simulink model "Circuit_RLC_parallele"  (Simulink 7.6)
settings: Solver=ode23t  StartTime=0.0  StopTime=0.05  RelTol=1e-3
InitFcn:
  | clc
  | clear all
  | delete *.mat
StopFcn:
  | close all
  | load circuit_RLC_parallele.mat
  | plot(x(1,:),x(2,:),x(1,:),x(3,:))
  | grid
  | title('Courant, tension - Circuit RLC parallèle')
  | xlabel('temps')
  | axis([0 0.05 -1 2])
libraries: powerlib x10

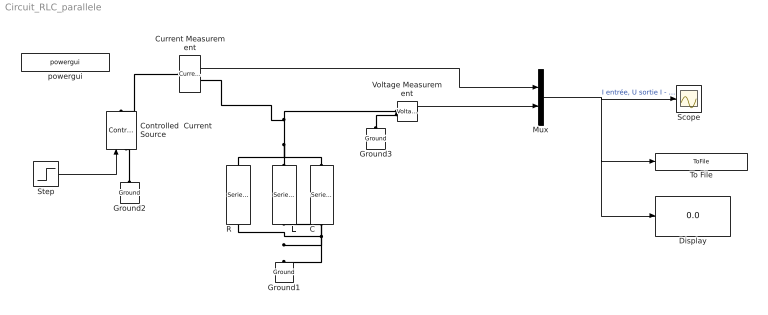
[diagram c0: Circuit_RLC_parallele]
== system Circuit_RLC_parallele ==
  C : powerlib/Elements/Series RLC Branch  DialogController=POWERSYS.PowerSysDialog  PhysicalDomain=powersysdomain  SubClassName=unknown  LeftPortType=p1  RightPortType=p1  LConnTagsString=__new0  RConnTagsString=__new0  BranchType=C  Resistance=1  Inductance=1e-3  SetiL0=off  InitialCurrent=0  Capacitance=0.001  Setx0=off  InitialVoltage=0  Measurements=None
  Controlled  Current Source : powerlib/Electrical Sources/Controlled Current Source  DialogController=POWERSYS.PowerSysDialog  SystemSampleTime=-1  Initialize=on  Source_Type=AC  Amplitude=0  Phase=0  Frequency=0  Measurements=None
  Current Measurement : powerlib/Measurements/Current Measurement  DialogController=POWERSYS.PowerSysDialog  SystemSampleTime=-1  PhasorSimulation=off  OutputType=Complex  PSBequivalent=0
  Display : Display
  Ground1 : powerlib/Elements/Ground  DialogController=POWERSYS.PowerSysDialog  PhysicalDomain=powersysdomain  SubClassName=unknown  LeftPortType=p1  RightPortType=p1  LConnTagsString=a
  Ground2 : powerlib/Elements/Ground  DialogController=POWERSYS.PowerSysDialog  PhysicalDomain=powersysdomain  SubClassName=unknown  LeftPortType=p1  RightPortType=p1  LConnTagsString=a
  Ground3 : powerlib/Elements/Ground  DialogController=POWERSYS.PowerSysDialog  PhysicalDomain=powersysdomain  SubClassName=unknown  LeftPortType=p1  RightPortType=p1  LConnTagsString=a
  L : powerlib/Elements/Series RLC Branch  DialogController=POWERSYS.PowerSysDialog  PhysicalDomain=powersysdomain  SubClassName=unknown  LeftPortType=p1  RightPortType=p1  LConnTagsString=__new0  RConnTagsString=__new0  BranchType=L  Resistance=4  Inductance=10e-3  SetiL0=off  InitialCurrent=0  Capacitance=0  Setx0=off  InitialVoltage=0  Measurements=None
  Mux : Mux  Inputs=2
  R : powerlib/Elements/Series RLC Branch  DialogController=POWERSYS.PowerSysDialog  PhysicalDomain=powersysdomain  SubClassName=unknown  LeftPortType=p1  RightPortType=p1  LConnTagsString=__new0  RConnTagsString=__new0  BranchType=R  Resistance=4  Inductance=10e-3  SetiL0=off  InitialCurrent=0  Capacitance=0  Setx0=off  InitialVoltage=0  Measurements=None
  Scope : Scope
  Step : Step  Time=0.005  SampleTime=0
  To File : ToFile  Filename=circuit_RLC_parallele  MatrixName=x
  Voltage Measurement : powerlib/Measurements/Voltage Measurement  DialogController=POWERSYS.PowerSysDialog  SystemSampleTime=-1  PhasorSimulation=off  OutputType=Complex  PSBequivalent=0
  powergui : powerlib/powergui  Priority=1  SystemSampleTime=-1  SimulationMode=Continuous  SampleTime=50e-6  frequency=60  SPID=off  DisableSnubberDevices=off  DisableRonSwitches=off  DisableVfSwitches=off  SwTol=0  Interpol=off  frequencyindice=0  echomessages=off  HookPort=off  DisplayEquations=off  FunctionMessages=off  EnableUseOfTLC=off  x0status=blocks  RestoreLinks=warning  ResistiveCurrentMeasurement=off  Frange=[0:2:500]  Ylog=off  Xlog=on  ShowGrid=on  save=off  variable=ZData  ZoomFFT=off  StartTime=0.0  cycles=1  DisplayStyle=1  fundamental=60  FreqAxis=off  MaxFrequency=1000  frequencyindicesteady=1  display=off  methode=off
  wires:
  Voltage Measurement/1 -> Mux/2
  Step/1 -> Controlled  Current Source/1
  Mux/1 -> Scope/1, To File/1, Display/1  "I entrée, U sortie I - RLC '//'"
  Current Measurement/1 -> Mux/1
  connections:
  Ground3/LConn1 -- Voltage Measurement/LConn2
  C/RConn1 -- R/LConn1 -- L/RConn1 -- Ground1/LConn1
  Current Measurement/LConn1 -- Controlled  Current Source/RConn1
  Ground2/LConn1 -- Controlled  Current Source/LConn1
  C/LConn1 -- Voltage Measurement/LConn1 -- Current Measurement/RConn1 -- R/RConn1 -- L/LConn1
